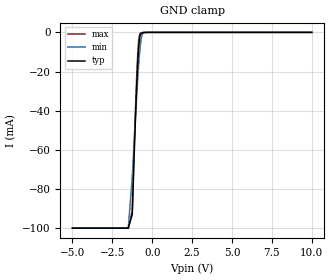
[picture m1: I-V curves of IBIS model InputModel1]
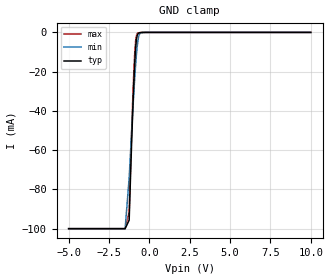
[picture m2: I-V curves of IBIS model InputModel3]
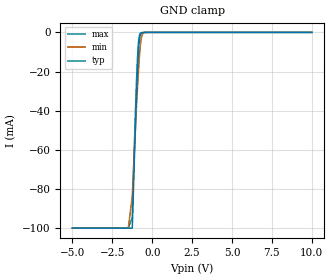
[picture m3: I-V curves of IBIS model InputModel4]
[IBIS Ver]   2.1
[File name]   e_016xs5.ibs   | e_= TSOP, f016xs= abbr chip name, 5= 5V Vcc
[File Rev]   2.40
[Date]   05-February-96
[Source]   File generated from lab measurements at Intel Corporation
[Notes]   Rev 2.00 fixes simulation model flaw.
   Rev 2.01 fixes typo errors in comments only.
   Rev 2.10 implements improvements for Quad parser IBIS2XTK:
   * adds zero current [POWER_clamp] to input models
   * changes model name from "I/O" to "InputOutput"
   * changes model type "Open_Drain" to "Open_drain"
   Rev 2.20 adds required dV/dt_r for OpenDrainOutput.
   Rev 2.30 adds 3/5# pin to pin #1.  The input model remains
   the same as it was included in rev 2.20, though the
   pin was a no connect in that model.
   Rev 2.40 All data was replaced by actual measurements
   performed in a lab.
[Disclaimer] INTEL DEVELOPER'S SOFTWARE LICENSE AGREEMENT
| BY USING THIS SOFTWARE, YOU ARE AGREEING TO BE BOUND
| BY THE TERMS OFTHIS AGREEMENT.  DO NOT USE THE SOFTWARE
| UNTIL YOU HAVE CAREFULLY READAND AGREED TO THE FOLLOWING
| TERMS AND CONDITIONS.  IF YOU DO NOT AGREETO THE TERMS
| OF THIS AGREEMENT, PROMPTLY RETURN THE SOFTWARE PACKAGE
| ANDANY ACCOMPANYING ITEMS.
| IF YOU USE THIS SOFTWARE, YOU WILL BE BOUND BY THE TERMS
| OF THIS AGREEMENT
| LICENSE: Intel Corporation ("Intel") grants you the non-exclusive right
| to use the enclosed software program ("Software").  You will not use,
| copy, modify, rent, sell or transfer the Software or any portion
| thereof, except as provided in this Agreement.
| System OEM Developers may:
| 1.   Copy the Software for support, backup or archival purposes;
| 2.   Install, use, or distribute Intel owned Software in object code
|   only;
| 3.   Modify and/or use Software source code that Intel directly makes
|   available to you as an OEM Developer;
| 4.   Install, use, modify, distribute, and/or make or have made
|   derivatives ("Derivatives") of Intel owned Software under the
|   terms and conditions in this Agreement, ONLY if you are a System
|   OEM Developer and NOT an end-user.
| RESTRICTIONS:
| YOU WILL NOT:
| 1.   Copy the Software, in whole or in part, except as provided for
|   in this Agreement;
| 2.   Decompile or reverse engineer any Software provided in object
|   code format;
| 3.   Distribute any Software or Derivative code to any end-users,
|   unless approved by Intel in a prior writing.
| TRANSFER: You may transfer the Software to another OEM
| Developer if thereceiving party agrees to the terms of this
| Agreement at the sole risk of any receiving party.
| OWNERSHIP AND COPYRIGHT OF SOFTWARE:
| Title to the Software and all copies thereof remain with Intel
| or its vendors.  The Software iscopyrighted and is protected by
| United States and international copyright laws.  You will not
| remove the copyright notice from the Software.  You agree to
| prevent any unauthorized copying of the Software.
| DERIVATIVE WORK: OEM Developers that make or have made
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[Copyright]   Copyright 1994,1996, Intel Corporation, All Rights Reserved
[Component]   E28F016XS   | 56-lead TSOP package, 28F016XS
[Manufacturer]  Intel   | Synchronous Flash Memory
|   | operating in 5V Vcc range
[Package]
| Variable   typ   min   max
|The following values apply for the Copper leadframe.
R_pkg   48m   41m   54m
L_pkg   4.92nH   4.44nH   5.39nH
C_pkg   0.48pF   0.45pF   0.50pF
|The following values apply for the Alloy-42 leadframe.
|R_pkg   195m   180m   210m
|L_pkg   4.92nH   4.44nH   5.39nH
|C_pkg   0.48pF   0.45pF   0.50pF
|*****************************Pin Definitions**********************************
[Pin]   signal_name   model_name   R_pin   L_pin   C_pin
  1   3/5#   InputModel1
  2   CE1#   InputModel1
  3   NC   InputModel2
  4   A20   InputModel3
  5   A19   InputModel3
  6   A18   InputModel1
  7   A17   InputModel1
  8   A16   InputModel1
  9   VCC   POWER
 10   A15   InputModel1
 11   A14   InputModel3
 12   A13   InputModel1
 13   A12   InputModel1
 14   CE0#   InputModel1
 15   VPP   POWER
 16   RP#   InputModel4
 17   A11   InputModel1
 18   A10   InputModel1
 19   A9   InputModel1
 20   A8   InputModel1
 21   GND   GND
 22   A7   InputModel1
 23   A6   InputModel1
 24   A5   InputModel1
 25   A4   InputModel1
 26   A3   InputModel1
 27   A2   InputModel1
 28   A1   InputModel1
 29   CLK   InputModel5
 30   ADV#   InputModel5
 31   BYTE#   InputModel1
 32   A0   InputModel1
 33   DQ0   InputOutput
 34   DQ8   InputOutput
 35   DQ1   InputOutput
 36   DQ9   InputOutput
 37   VCC   POWER
 38   DQ2   InputOutput
 39   DQ10   InputOutput
 40   DQ3   InputOutput
 41   DQ11   InputOutput
 42   GND   GND
 43   VCC   POWER
 44   DQ4   InputOutput
 45   DQ12   InputOutput
 46   DQ5   InputOutput
 47   DQ13   InputOutput
 48   GND   GND
 49   DQ6   InputOutput
 50   DQ14   InputOutput
 51   DQ7   InputOutput
 52   DQ15   InputOutput
 53   RY/BY#   OpenDrainOutput
 54   OE#   InputModel1
 55   WE#   InputModel4
 56   WP#   InputModel1
|**********************Input Model 2************************************
[Model]   InputModel2
Model_type   Input
|   for pin3(NC)
Vinl = 0.8V
Vinh = 2.0V
| Variable   typ   min   max
C_comp   5.61p   NA   7.6p
[Voltage Range]   5.0V   4.5V   5.5V
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| Models and submodels in the file (7): InputModel1 (Input), InputModel2 (Input), InputModel3 (Input), InputModel4 (Input), InputModel5 (Input), InputOutput (I/O), OpenDrainOutput (Open_drain)
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|**************************Input Model 1***************************************
[Model]   InputModel1
Model_type   Input
|   for pin1(3/5#), CE1#, CE0#, OE#, WP#, BYTE#, A[18:15], A[13:0]
Vinl = 0.8V
Vinh = 2.0V
| Variable   typ   min   max
C_comp   5.61p   NA   7.6p
[Voltage Range]   5.0V   4.5V   5.5V
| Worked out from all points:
|   GND clamp passes 1 mA (typ) near -0.73 V on its own axis
[GND_clamp]
|Voltage I(typ)   I(min)   I(max)
-5V       -99.95mA   -99.95mA   -99.95mA
-1.5V     -99.95mA   -99.95mA   -99.95mA
-1.25V    -92.96mA   -74.04mA   -90.95mA
-1.1V     -55.65mA   -51.01mA   -51.19mA
-1V       -33.11mA   -36.32mA   -27.73mA
-950mV    -23.17mA   -29.39mA   -17.78mA
-900mV    -14.53mA   -22.64mA   -9.695mA
-850mV    -7.833mA   -16.49mA   -4.184mA
-750mV    -1.35mA    -7.041mA   -521.9uA
-650mV    -265.4uA   -1.784mA   -152.7uA
-500mV    -44.52uA   -116.6uA   -16.83uA
10V       0A         0A         0A
[POWER_clamp]
| Input buffer circuits of this product do not intrinsically
| require a [POWER_clamp] definition.  This zero current
| [POWER_clamp] is provided for compatibility with some ibis
| parsers.
|   Voltage  I(typ)   I(min)   I(max)
-5V       0A         0A         0A
-4.75V    0A         0A         0A
9.75V     0A         0A         0A
10V       0A         0A         0A
|*********************Input Model 3**************************************
[Model]   InputModel3
Model_type   Input
|   for A[20], A[19], A[14]
Vinl = 0.8V
Vinh = 2.0V
| Variable   typ   min   max
C_comp   5.61p   NA   7.6p
[Voltage Range]   5.0V   4.5V   5.5V
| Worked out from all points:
|   GND clamp passes 1 mA (typ) near -0.72 V on its own axis
[GND_clamp]
|Voltage I(typ)   I(min)   I(max)
-5V       -99.95mA   -99.95mA   -99.95mA
-1.5V     -99.95mA   -99.95mA   -99.95mA
-1.25V    -95.61mA   -74.11mA   -91.28mA
-1.1V     -56.86mA   -50.87mA   -51mA
-1V       -33.64mA   -36.12mA   -27.59mA
-950mV    -23.47mA   -29.17mA   -17.64mA
-900mV    -14.69mA   -22.58mA   -9.632mA
-850mV    -7.929mA   -16.55mA   -4.193mA
-750mV    -1.418mA   -6.928mA   -582.8uA
-650mV    -309.5uA   -1.797mA   -190.1uA
-500mV    -55.99uA   -137.2uA   -23.18uA
10V       0A         0A         0A
[POWER_clamp]
| Input buffer circuits of this product do not intrinsically
| require a [POWER_clamp] definition.  This zero current
| [POWER_clamp] is provided for compatibility with some ibis
| parsers.
|   Voltage  I(typ)   I(min)   I(max)
-5V       0A         0A         0A
-4.75V    0A         0A         0A
9.75V     0A         0A         0A
10V       0A         0A         0A
|**********************Input Model 4***************************************
[Model]   InputModel4
Model_type   Input
|   for RP#, WE#
Vinl = 0.8V
Vinh = 2.0V
| Variable   typ   min   max
C_comp   5.61p   NA   7.6p
[Voltage Range]   5.0V   4.5V   5.5V
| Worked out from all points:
|   GND clamp passes 1 mA (typ) near -0.73 V on its own axis
[GND_clamp]
|Voltage I(typ)   I(min)   I(max)
-5V       -99.95mA   -99.95mA   -99.95mA
-1.5V     -99.95mA   -99.95mA   -99.95mA
-1.25V    -99.95mA   -83.71mA   -94.58mA
-1.1V     -60.17mA   -57.48mA   -52.75mA
-1V       -35.39mA   -40.15mA   -28.2mA
-950mV    -24.54mA   -32.57mA   -17.85mA
-900mV    -15.18mA   -25.02mA   -9.577mA
-850mV    -8.031mA   -18.13mA   -4.078mA
-750mV    -1.321mA   -7.097mA   -514.4uA
-650mV    -215.8uA   -1.753mA   -148uA
-500mV    -23.9uA    -122.1uA   -15.49uA
10V       0A         0A         0A
[POWER_clamp]
| Input buffer circuits of this product do not intrinsically
| require a [POWER_clamp] definition.  This zero current
| [POWER_clamp] is provided for compatibility with some ibis
| parsers.
|   Voltage  I(typ)   I(min)   I(max)
-5V       0A         0A         0A
-4.75V    0A         0A         0A
9.75V     0A         0A         0A
10V       0A         0A         0A
